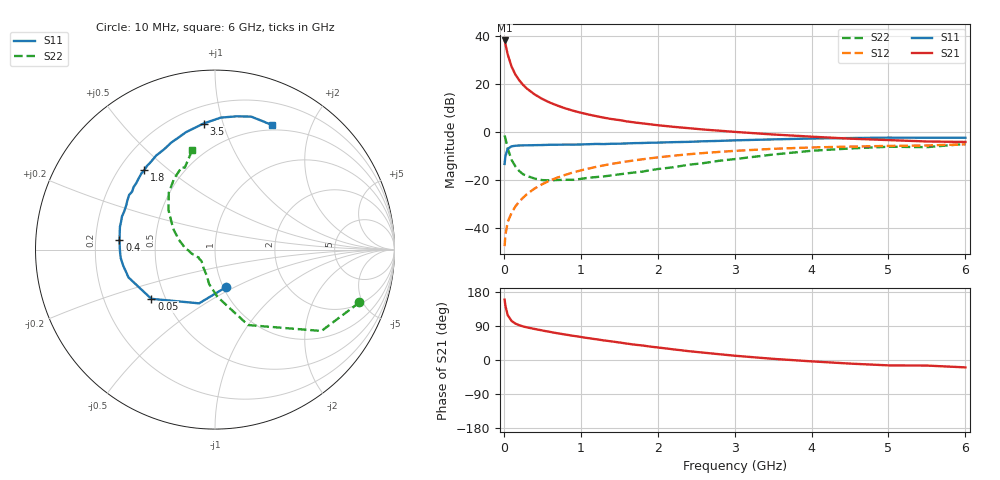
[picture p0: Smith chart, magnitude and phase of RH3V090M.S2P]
! SIEMENS Small Signal Semiconductors
! BFR106
! Si NPN RF Bipolar Junction Transistor in SOT23
! VCE = 3 V  IC = 90 mA
! Common Emitter S-Parameters:  August  1996
# GHz  S  MA  R  50
!  f  S11  S21  S12  S22
! GHz  MAG  ANG  MAG  ANG  MAG  ANG  MAG  ANG
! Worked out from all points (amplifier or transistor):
!   36 points, 10 MHz to 6 GHz, reference 50 ohm
!   highest |S21| = 38.2 dB at 10 MHz (marker M1)
!   |S21| within 3 dB of that: start of sweep to 31.21 MHz
!   unconditionally stable (mu >= 1): 167.7 MHz to 2.599 GHz; 5.341 GHz to end of sweep
!   at 250 MHz: K = 1.07, MAG = 21.9 dB, |S12| = -27.3 dB
!   at 1.4 GHz: K = 1.07, MAG = 7.8 dB, |S12| = -13.3 dB
!   at 6 GHz: K = 1.01, MAG = 0.0 dB, |S12| = -5.1 dB
!   S11 on the Smith chart (normalised r, x): 10 MHz: 1.03, -0.45; 50 MHz: 0.42, -0.29; 400 MHz: 0.30, +0.05; 1.8 GHz: 0.30, +0.42; 3.5 GHz: 0.31, +0.86; 6 GHz: 0.44, +1.47
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0.01  0.2176 -73.1  81.31 159.5  0.0042 77.2  0.857 -20.1
0.02  0.3123 -106.5  69.7 143.6  0.0071 69.9  0.7465 -37.4
0.05  0.4484 -142.3  41.77 118.3  0.0134 61.5  0.4592 -66.3
0.1  0.506 -162.1  23.3 103.2  0.0206 66.1  0.2639 -87.0
0.15  0.5195 -170.2  15.85 96.1  0.0282 69.1  0.1938 -99.9
0.2  0.5273 -174.9  12.07 91.9  0.0357 72.2  0.1549 -106.7
0.25  0.5291 -178.4  9.643 88.5  0.043 72.6  0.1324 -115.3
0.3  0.5308 178.8  8.079 86.2  0.051 73.7  0.1225 -120.8
0.4  0.5349 174.2  6.11 81.9  0.0669 73.7  0.1075 -130.8
0.5  0.5382 170.6  4.906 77.9  0.0823 73.3  0.1 -137.8
0.6  0.5447 166.5  4.113 74.2  0.0981 72.5  0.0989 -141.9
0.7  0.5461 163.3  3.553 70.4  0.1135 71.3  0.1006 -146.8
0.9  0.5487 157.3  2.794 63.9  0.1444 68.5  0.1012 -154.9
1.1  0.5596 150.8  2.327 57.6  0.1737 65.6  0.112 -160.0
1.4  0.5718 142.5  1.874 49.1  0.2171 60.8  0.1253 -167.9
1.8  0.593 131.5  1.52 38.3  0.2713 54.2  0.1501 -178.7
2.2  0.6178 122.1  1.291 28.2  0.322 47.7  0.1851 170.6
2.8  0.6563 108.1  1.071 15.3  0.3871 37.8  0.253 154.8
3.5  0.7054 95.2  0.893 3.1  0.4489 26.9  0.3411 139.5
4.5  0.752 80.9  0.731 -9.5  0.4987 12.4  0.4559 120.0
5.5  0.7631 69.0  0.638 -14.7  0.5273 3.4  0.4862 110.3
6  0.7625 65.2  0.624 -19.5  0.5571 -3.5  0.5671 103.0
